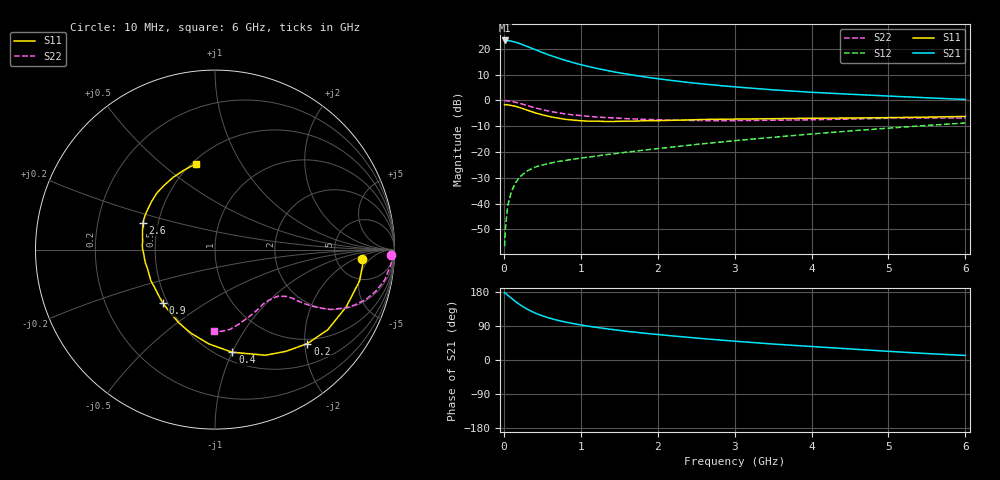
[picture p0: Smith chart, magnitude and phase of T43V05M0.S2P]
! Infineon Technologies  Discrete & RF Semiconductors
! BFR182T
! Si NPN RF Bipolar Junction Transistor in SC75
! VCE = 3 V  IC = 5 mA
! Common Emitter S-Parameters:  October  1999
# GHz  S  MA  R  50
!  f  S11  S21  S12  S22
! GHz  MAG  ANG  MAG  ANG  MAG  ANG  MAG  ANG
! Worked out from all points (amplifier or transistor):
!   36 points, 10 MHz to 6 GHz, reference 50 ohm
!   highest |S21| = 23.3 dB at 10 MHz (marker M1)
!   |S21| within 3 dB of that: start of sweep to 361.4 MHz
!   unconditionally stable (mu >= 1): 1.385 GHz to 4.023 GHz
!   at 250 MHz: K = 0.28, MSG = 25.1 dB, |S12| = -28.6 dB
!   at 1.4 GHz: K = 1.01, MAG = 15.6 dB, |S12| = -20.8 dB
!   at 6 GHz: K = 0.84, MSG = 4.6 dB, |S12| = -8.7 dB
!   lowest NFmin = 1.20 dB at 450 MHz
!   S11 on the Smith chart (normalised r, x): 10 MHz: 9.27, -2.85; 200 MHz: 0.90, -2.05; 400 MHz: 0.58, -1.00; 900 MHz: 0.47, -0.34; 2.6 GHz: 0.41, +0.15; 6 GHz: 0.52, +0.66
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0.01  0.8207 -3.5  14.54 177.4  0.0015 77.4  0.9838 -1.8
0.02  0.8305 -3.6  14.52 176.6  0.0032 83.7  0.9958 -2.2
0.05  0.8243 -12.2  14.49 171.0  0.0091 87.8  0.982 -5.2
0.1  0.7976 -23.6  14.06 162.8  0.0175 79.3  0.9603 -10.2
0.15  0.771 -35.4  13.5 154.5  0.025 72.1  0.9245 -14.6
0.2  0.7341 -45.5  12.81 147.1  0.032 69.1  0.8854 -18.3
0.25  0.6915 -55.0  11.99 140.5  0.0373 64.0  0.8406 -21.4
0.3  0.6525 -64.4  11.2 134.5  0.0427 61.6  0.8 -23.9
0.4  0.5802 -80.4  9.765 124.4  0.0508 56.7  0.7232 -27.5
0.5  0.5263 -93.8  8.515 116.6  0.056 54.3  0.6636 -29.2
0.6  0.4852 -105.8  7.477 110.1  0.0607 52.4  0.6158 -30.5
0.7  0.4555 -116.3  6.662 104.8  0.0654 52.0  0.5778 -31.2
0.8  0.4308 -125.4  5.99 100.1  0.0689 52.1  0.5484 -31.7
0.9  0.4167 -134.1  5.41 96.2  0.0725 52.4  0.5244 -32.0
1.1  0.3969 -148.3  4.549 89.0  0.0799 53.5  0.4924 -32.7
1.6  0.3965 -173.5  3.237 75.7  0.0997 56.4  0.4436 -35.6
2.2  0.4127 168.5  2.419 63.4  0.1255 59.7  0.417 -41.5
2.6  0.4282 159.4  2.079 56.2  0.1455 61.1  0.4068 -46.2
3.5  0.4431 143.4  1.605 42.1  0.1933 61.4  0.4138 -58.0
4.5  0.4563 128.6  1.32 29.2  0.2562 59.0  0.4362 -72.4
5.5  0.4753 111.1  1.126 17.0  0.328 54.4  0.457 -85.5
6  0.4903 102.6  1.044 12.0  0.3661 51.0  0.4555 -91.0
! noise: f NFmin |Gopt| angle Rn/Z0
0.45  1.2  0.27  37  0.3
0.9  1.3  0.25  75  0.23
1.8  1.9  0.21  145  0.2
